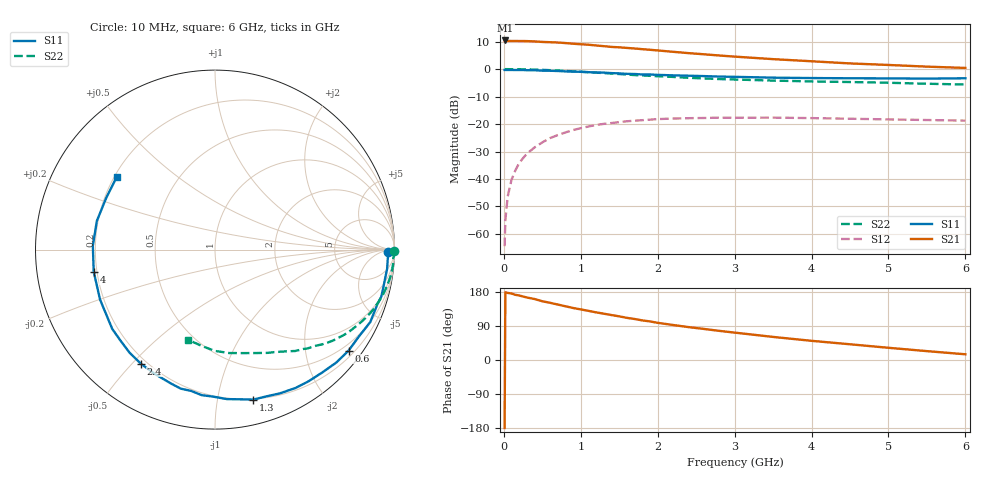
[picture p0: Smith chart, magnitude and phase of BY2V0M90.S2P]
! SIEMENS Small Signal Semiconductors
! BFY420
! Si NPN RF SIEGET Grounded Emitter Transistor in MICRO-X
! VCE = 2 V  IC = 0.9 mA
! Common Emitter S-Parameters:  October  1996
# GHz  S  MA  R  50
!  f  S11  S21  S12  S22
! GHz  MAG  ANG  MAG  ANG  MAG  ANG  MAG  ANG
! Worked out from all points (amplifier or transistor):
!   36 points, 10 MHz to 6 GHz, reference 50 ohm
!   highest |S21| = 10.4 dB at 20 MHz (marker M1)
!   |S21| within 3 dB of that: start of sweep to 1.732 GHz
!   unconditionally stable (mu >= 1): 4.581 GHz to end of sweep
!   at 250 MHz: K = 0.03, MSG = 21.3 dB, |S12| = -32.4 dB
!   at 1.4 GHz: K = 0.20, MSG = 13.8 dB, |S12| = -19.6 dB
!   at 6 GHz: K = 1.35, MAG = 6.1 dB, |S12| = -18.7 dB
!   S11 on the Smith chart (normalised r, x): 10 MHz: 49, -19; 600 MHz: 0.34, -2.95; 1.3 GHz: 0.19, -1.27; 2.4 GHz: 0.18, -0.53; 4 GHz: 0.19, -0.09; 6 GHz: 0.21, +0.32
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0.01  0.9653 -0.8  3.3 -179.4  0.0006 109.7  0.9987 -0.3
0.02  0.9655 -1.3  3.319 178.8  0.0018 82.8  0.9979 -0.5
0.05  0.9638 -3.4  3.254 177.0  0.0048 88.0  0.9976 -1.6
0.1  0.9649 -6.4  3.245 175.5  0.0097 86.8  0.9938 -3.1
0.15  0.9615 -9.4  3.245 172.0  0.0144 83.2  0.9955 -4.7
0.2  0.9614 -12.6  3.241 170.2  0.0196 83.5  0.9938 -6.1
0.3  0.9546 -18.5  3.231 164.9  0.0289 78.7  0.9877 -9.2
0.4  0.9548 -25.0  3.191 160.9  0.0376 75.1  0.9789 -12.2
0.5  0.9366 -31.1  3.12 155.0  0.0464 71.1  0.9687 -15.2
0.6  0.9331 -37.1  3.085 151.0  0.0555 67.5  0.9558 -18.0
0.8  0.9089 -48.8  2.977 141.8  0.0703 59.8  0.927 -23.6
1.1  0.8788 -65.7  2.778 129.7  0.0903 50.2  0.8781 -31.1
1.3  0.8625 -75.7  2.613 122.2  0.1008 44.3  0.8454 -35.5
1.7  0.8143 -95.2  2.371 108.2  0.1152 33.8  0.7782 -43.4
2.2  0.7696 -115.9  2.063 92.4  0.1259 23.1  0.7199 -51.7
2.4  0.7582 -123.1  1.952 86.8  0.1279 19.8  0.6944 -54.7
2.8  0.7309 -136.1  1.767 76.9  0.1307 13.6  0.6585 -60.2
3.5  0.6983 -156.5  1.517 60.9  0.1309 5.5  0.6178 -68.9
4  0.6869 -169.7  1.388 50.6  0.1283 1.2  0.596 -75.4
4.5  0.6809 178.2  1.268 41.5  0.1249 -2.3  0.5816 -82.2
5.5  0.6711 154.5  1.108 23.4  0.1184 -5.2  0.5415 -98.0
6  0.6807 143.6  1.05 15.1  0.1155 -4.8  0.5238 -106.8
